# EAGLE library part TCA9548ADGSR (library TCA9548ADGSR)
Switch ICs - Various 8-channel 1.65- to 5 .5-V I2C/SMBus switc Source: Datasheet
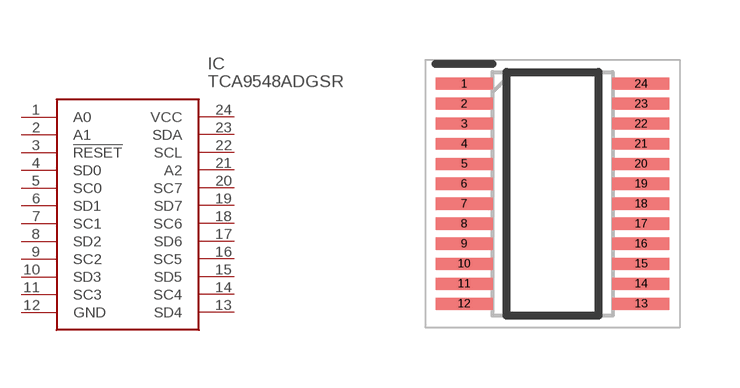
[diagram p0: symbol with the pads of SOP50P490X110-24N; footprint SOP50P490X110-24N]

Designator prefix IC

## TCA9548ADGSR (Arrow_Part_Number: TCA9548ADGSR; Arrow_Price-Stock: https://www.arrow.com/en/products/tca9548adgsr/texas-instruments.html?utm_currency=USD&region=nac; Description: Switch ICs - Various 8-channel 1.65- to 5 .5-V I2C/SMBus switc; Height: 1.1mm; Manufacturer_Name: Texas Instruments; Manufacturer_Part_Number: TCA9548ADGSR; Mouser_Part_Number: 595-TCA9548ADGSR; Mouser_Price-Stock: https://www.mouser.co.uk/ProductDetail/Texas-Instruments/TCA9548ADGSR?qs=olJun0bQHM%252B7USbLxm4jDw%3D%3D)  [SOP50P490X110-24N]
1  A0
2  A1
3  !RESET
4  SD0
5  SC0
6  SD1
7  SC1
8  SD2
9  SC2
10  SD3
11  SC3
12  GND
13  SD4
14  SC4
15  SD5
16  SC5
17  SD6
18  SC6
19  SD7
20  SC7
21  A2
22  SCL
23  SDA
24  VCC

## Footprint SOP50P490X110-24N (pad centres in mm)
DGS0024A
smd 1.425 x 0.3: 1 -2.212,2.75; 2 -2.212,2.25; 3 -2.212,1.75; 4 -2.212,1.25; 5 -2.212,0.75; 6 -2.212,0.25; 7 -2.212,-0.25; 8 -2.212,-0.75; 9 -2.212,-1.25; 10 -2.212,-1.75; 11 -2.212,-2.25; 12 -2.212,-2.75; 13 2.212,-2.75; 14 2.212,-2.25; 15 2.212,-1.75; 16 2.212,-1.25; 17 2.212,-0.75; 18 2.212,-0.25; 19 2.212,0.25; 20 2.212,0.75; 21 2.212,1.25; 22 2.212,1.75; 23 2.212,2.25; 24 2.212,2.75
